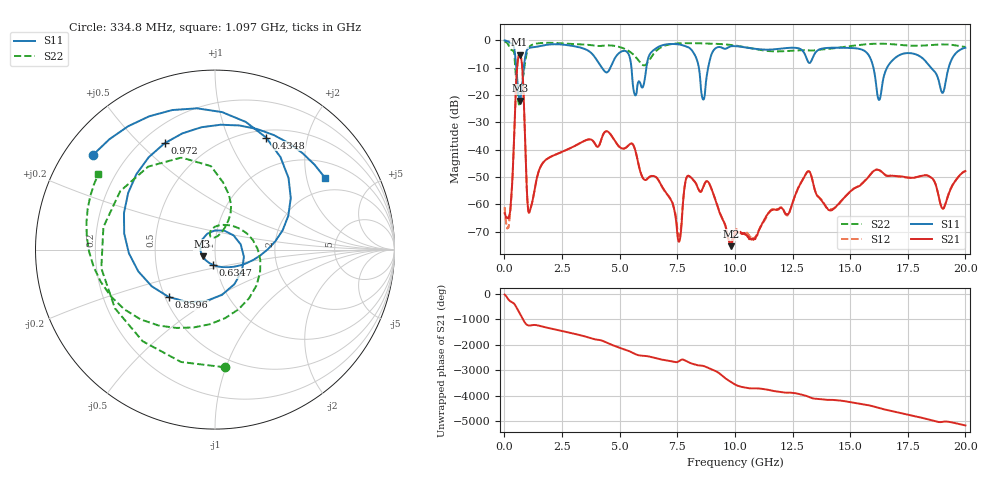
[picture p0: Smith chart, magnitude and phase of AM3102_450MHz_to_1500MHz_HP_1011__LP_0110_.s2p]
!Agilent Technologies,E8364B,MY43040894,A.07.50.67
!Agilent E8364B: A.07.50.67
!Date: Thursday, January 11, 2018 06:24:25
!Correction: S11(Full 2 Port(1,2))
!S21(Full 2 Port(1,2))
!S12(Full 2 Port(1,2))
!S22(Full 2 Port(1,2))
!S2P File: Measurements: S11, S21, S12, S22:
# Hz S  dB  R 50
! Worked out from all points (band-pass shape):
!   1601 points, 10 MHz to 20 GHz, reference 50 ohm
!   highest |S21| = -5.28 dB at 659.7 MHz (marker M1); lowest = -75.3 dB at 9.818 GHz (marker M2)
!   |S21| within 3 dB of the highest: 571 MHz to 757.5 MHz (186.5 MHz wide, 28.1 % of centre)
!   lowest |S11| = -22.1 dB at 672.2 MHz (marker M3), VSWR 1.17, Z = 43.4 - j3.22 ohm
!   |S11| at or under -10 dB: 5.513 GHz to 6.159 GHz (645.7 MHz wide, 11.1 % of centre); 16.01 GHz to 16.6 GHz (591.1 MHz wide, 3.63 % of centre); 18.51 GHz to 19.27 GHz (767.2 MHz wide, 4.06 % of centre)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
!   |S22| runs from -23.5 to -0.4 dB; largest |S21 - S12| = 0.00083
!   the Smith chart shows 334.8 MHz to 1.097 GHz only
!   S11 on the Smith chart (normalised r, x): 334.8 MHz: 0.08, +0.34; 434.8 MHz: 0.59, +1.38; 634.7 MHz: 0.96, -0.17; 859.6 MHz: 0.52, -0.32; 972 MHz: 0.29, +0.59; 1.097 GHz: 1.49, +2.57
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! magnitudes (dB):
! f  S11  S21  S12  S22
! 10 MHz  -0.1  -63.2  -61.0  -0.4
! 334.8 MHz  -1.3  -52.8  -53.0  -3.6
! 434.8 MHz  -3.3  -31.9  -32.1  -5.3
! 634.7 MHz  -21.3  -5.4  -5.4  -23.5
! 659.7 MHz  -22.1  -5.3  -5.3  -22.6
! 672.2 MHz  -22.1  -5.4  -5.4  -21.4
! 859.6 MHz  -8.7  -26.2  -26.3  -10.3
! 972 MHz  -3.7  -54.3  -54.2  -4.4
! 1.097 GHz  -2.7  -62.6  -62.3  -2.2
! 3.346 GHz  -2.8  -37.3  -37.3  -1.5
! 5.295 GHz  -4.1  -39.1  -39.1  -3.4
! 5.682 GHz  -20.1  -40.3  -40.3  -6.0
! 6.682 GHz  -2.4  -51.1  -51.1  -3.2
! 7.581 GHz  -1.5  -73.6  -71.6  -1.1
! 7.931 GHz  -2.4  -49.7  -49.8  -1.0
! 8.618 GHz  -21.6  -53.8  -53.7  -1.1
! 9.818 GHz  -2.2  -75.3  -73.6  -1.7
! 10.01 GHz  -2.1  -71.2  -70.0  -1.9
! 13.34 GHz  -7.1  -50.3  -50.4  -3.7
! 16.68 GHz  -8.9  -49.6  -49.5  -1.3
! 19.01 GHz  -19.2  -61.5  -61.6  -1.5
! 20 GHz  -2.7  -47.8  -47.9  -2.4
